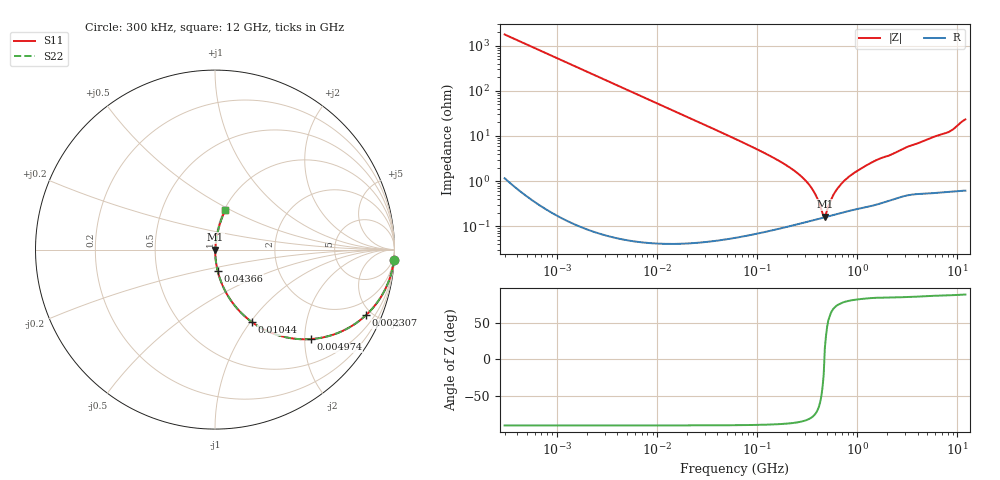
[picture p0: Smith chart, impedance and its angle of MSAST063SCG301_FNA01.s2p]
! MSAST063SCG301_FNA01  S-PARAMETER MODEL  ( General Type )
! Model Generated by TAIYO YUDEN Corporation (http://www.ty-top.com)
! Version 1.0
! TAIYO YUDEN Control No. 160830
! Copyright(c) 2016 TAIYO YUDEN CO.,LTD. All Rights Reserved.
! Product Description (link to TY-COMPAS)
! https://ds.yuden.co.jp/TYCOMPAS/or/detail?pn=MSAST063SCG301JFNA01&u=M
! Products Name : Multilayer Ceramic Capacitors
! Characteristics :
!  Capacitance : 300 pF , Rated Voltage : 25V , TCC : CG / C0G
!  Case Size : 0.6 x 0.3 / 0.024 x 0.012 [mm/inch] , Thickness : 0.3 / 0.012 [mm/inch]
!  (Conditions: Temperature = 25 degC , DC Bias Current/Voltage = 0A / 0V)
! External Node Assignments :
!  1  o---| |---o  2
! GND o---------o GND
! Frequency Range : 0.3MHz  -  12000MHz  [ 401 STEP ]
# MHz S RI R 50
! Freq[MHz].  S11 Real  S11 Imag  S21 Real  S21 Imag  S12 Real  S12 Imag  S22 Real  S22 Imag
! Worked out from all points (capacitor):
!   401 points, 300 kHz to 12 GHz, reference 50 ohm
!   read as one part in series: C = 300 pF near 316.3 kHz
!   lowest |Z| = 165 mohm at 473.8 MHz (marker M1)
!   series resonance near 468.4 MHz, so ESL is about 380 pH
!   S11 on the Smith chart (normalised r, x): 300 kHz: 1, -35; 2.307 MHz: 1.00, -4.60; 4.974 MHz: 1.00, -2.13; 10.44 MHz: 1.00, -1.02; 43.66 MHz: 1.00, -0.24; 12 GHz: 1.01, +0.47
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0.3  0.9968 -0.0564  0.00322 0.0564  0.00322 0.0564  0.9968 -0.0564
0.778586  0.9789 -0.1437  0.0211 0.1437  0.0211 0.1437  0.9789 -0.1437
1.769972  0.8998 -0.3002  0.1002 0.3002  0.1002 0.3002  0.8998 -0.3002
2.306842  0.8409 -0.3656  0.1591 0.3656  0.1591 0.3656  0.8409 -0.3656
4.973558  0.5322 -0.4987  0.4678 0.4987  0.4678 0.4987  0.5322 -0.4987
10.44266  0.2052 -0.4034  0.7948 0.4034  0.7948 0.4034  0.2052 -0.4034
19.20568  0.071 -0.2561  0.929 0.2561  0.929 0.2561  0.071 -0.2561
43.66058  0.0148 -0.1186  0.9852 0.1186  0.9852 0.1186  0.0148 -0.1186
60  0.00806 -0.0863  0.9919 0.0863  0.9919 0.0863  0.00806 -0.0863
202.9496  0.00144 -0.0213  0.9986 0.0213  0.9986 0.0213  0.00144 -0.0213
278.9009  0.00133 -0.0124  0.9987 0.0124  0.9987 0.0124  0.00133 -0.0124
353.9943  0.00139 -0.0066  0.9986 0.0066  0.9986 0.0066  0.00139 -0.0066
393.5654  0.00145 -0.00417  0.9986 0.00417  0.9986 0.00417  0.00145 -0.00417
449.3064  0.00154 -0.00118  0.9985 0.00118  0.9985 0.00118  0.00154 -0.00118
473.7541  0.00159 0.000445  0.9984 -0.000445  0.9984 -0.000445  0.00159 0.000445
585.5907  0.00182 0.00498  0.9982 -0.00498  0.9982 -0.00498  0.00182 0.00498
763.2128  0.00221 0.0106  0.9978 -0.0106  0.9978 -0.0106  0.00221 0.0106
1296.429  0.0033 0.0236  0.9967 -0.0236  0.9967 -0.0236  0.0033 0.0236
2088.533  0.00506 0.0368  0.9949 -0.0368  0.9949 -0.0368  0.00506 0.0368
3190.978  0.00815 0.0571  0.9919 -0.0571  0.9919 -0.0571  0.00815 0.0571
8064.993  0.02 0.1181  0.98 -0.1181  0.98 -0.1181  0.02 0.1181
12000  0.0567 0.2183  0.9433 -0.2183  0.9433 -0.2183  0.0567 0.2183
